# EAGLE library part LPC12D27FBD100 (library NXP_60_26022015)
LPC12D27 32-bit ARM Cortex-M0 microcontroller; 128 kB flash and 8 kB SRAM; 40 segment x 4 LCD driver AAL Eindhoven MK
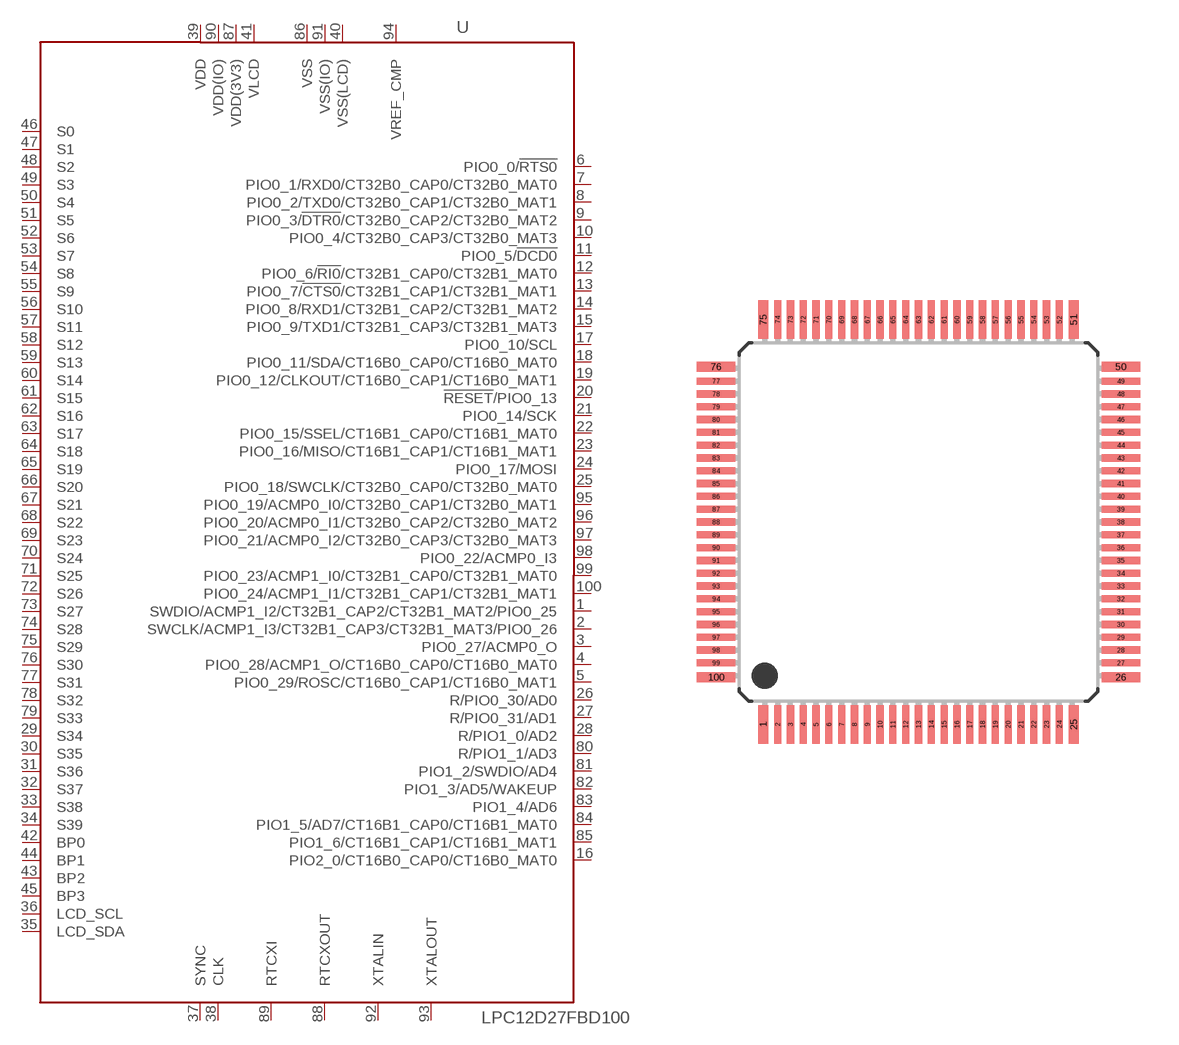
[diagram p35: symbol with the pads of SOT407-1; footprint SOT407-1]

Designator prefix U

## LPC12D27FBD100  [SOT407-1]
1  SWDIO/ACMP1_I2/CT32B1_CAP2/CT32B1_MAT2/PIO0_25
2  SWCLK/ACMP1_I3/CT32B1_CAP3/CT32B1_MAT3/PIO0_26
3  PIO0_27/ACMP0_O
4  PIO0_28/ACMP1_O/CT16B0_CAP0/CT16B0_MAT0
5  PIO0_29/ROSC/CT16B0_CAP1/CT16B0_MAT1
6  PIO0_0/!RTS0!
7  PIO0_1/RXD0/CT32B0_CAP0/CT32B0_MAT0
8  PIO0_2/TXD0/CT32B0_CAP1/CT32B0_MAT1
9  PIO0_3/!DTR0!/CT32B0_CAP2/CT32B0_MAT2
10  PIO0_4/CT32B0_CAP3/CT32B0_MAT3
11  PIO0_5/!DCD0!
12  PIO0_6/!RI0!/CT32B1_CAP0/CT32B1_MAT0
13  PIO0_7/!CTS0!/CT32B1_CAP1/CT32B1_MAT1
14  PIO0_8/RXD1/CT32B1_CAP2/CT32B1_MAT2
15  PIO0_9/TXD1/CT32B1_CAP3/CT32B1_MAT3
16  PIO2_0/CT16B0_CAP0/CT16B0_MAT0
17  PIO0_10/SCL
18  PIO0_11/SDA/CT16B0_CAP0/CT16B0_MAT0
19  PIO0_12/CLKOUT/CT16B0_CAP1/CT16B0_MAT1
20  !RESET!/PIO0_13
21  PIO0_14/SCK
22  PIO0_15/SSEL/CT16B1_CAP0/CT16B1_MAT0
23  PIO0_16/MISO/CT16B1_CAP1/CT16B1_MAT1
24  PIO0_17/MOSI
25  PIO0_18/SWCLK/CT32B0_CAP0/CT32B0_MAT0
26  R/PIO0_30/AD0
27  R/PIO0_31/AD1
28  R/PIO1_0/AD2
29  S34  out
30  S35  out
31  S36  out
32  S37  out
33  S38  out
34  S39  out
35  LCD_SDA
36  LCD_SCL
37  SYNC
38  CLK
39  VDD  pwr
40  VSS(LCD)  pwr
41  VLCD  pwr
42  BP0  out
43  BP2  out
44  BP1  out
45  BP3  out
46  S0  out
47  S1  out
48  S2  out
49  S3  out
50  S4  out
51  S5  out
52  S6  out
53  S7  out
54  S8  out
55  S9  out
56  S10  out
57  S11  out
58  S12  out
59  S13  out
60  S14  out
61  S15  out
62  S16  out
63  S17  out
64  S18  out
65  S19  out
66  S20  out
67  S21  out
68  S22  out
69  S23  out
70  S24  out
71  S25  out
72  S26  out
73  S27  out
74  S28  out
75  S29  out
76  S30  out
77  S31  out
78  S32  out
79  S33  out
80  R/PIO1_1/AD3
81  PIO1_2/SWDIO/AD4
82  PIO1_3/AD5/WAKEUP
83  PIO1_4/AD6
84  PIO1_5/AD7/CT16B1_CAP0/CT16B1_MAT0
85  PIO1_6/CT16B1_CAP1/CT16B1_MAT1
86  VSS  pwr
87  VDD(3V3)  pwr
88  RTCXOUT  pas
89  RTCXI  pas
90  VDD(IO)  pwr
91  VSS(IO)  pwr
92  XTALIN  pas
93  XTALOUT  pas
94  VREF_CMP  pwr
95  PIO0_19/ACMP0_I0/CT32B0_CAP1/CT32B0_MAT1
96  PIO0_20/ACMP0_I1/CT32B0_CAP2/CT32B0_MAT2
97  PIO0_21/ACMP0_I2/CT32B0_CAP3/CT32B0_MAT3
98  PIO0_22/ACMP0_I3
99  PIO0_23/ACMP1_I0/CT32B1_CAP0/CT32B1_MAT0
100  PIO0_24/ACMP1_I1/CT32B1_CAP1/CT32B1_MAT1

## Footprint SOT407-1 (pad centres in mm)
SOT407-1 LQFP100: plastic low profile quad flat package; 100 leads; body 14 x 14 x 1.4 mm JEDEC: MS-026 IEC: 136E20
smd 0.4 x 1.5: 1 -6.06,-7.9; 25 6.06,-7.9; 51 6.06,7.9; 75 -6.06,7.9
smd 0.28 x 1.5: 2 -5.5,-7.9; 3 -5,-7.9; 4 -4.5,-7.9; 5 -4,-7.9; 6 -3.5,-7.9; 7 -3,-7.9; 8 -2.5,-7.9; 9 -2,-7.9; 10 -1.5,-7.9; 11 -1,-7.9; 12 -0.5,-7.9; 13 0,-7.9; 14 0.5,-7.9; 15 1,-7.9; 16 1.5,-7.9; 17 2,-7.9; 18 2.5,-7.9; 19 3,-7.9; 20 3.5,-7.9; 21 4,-7.9; 22 4.5,-7.9; 23 5,-7.9; 24 5.5,-7.9; 52 5.5,7.9; 53 5,7.9; 54 4.5,7.9; 55 4,7.9; 56 3.5,7.9; 57 3,7.9; 58 2.5,7.9; 59 2,7.9; 60 1.5,7.9; 61 1,7.9; 62 0.5,7.9; 63 0,7.9; 64 -0.5,7.9; 65 -1,7.9; 66 -1.5,7.9; 67 -2,7.9; 68 -2.5,7.9; 69 -3,7.9; 70 -3.5,7.9; 71 -4,7.9; 72 -4.5,7.9; 73 -5,7.9; 74 -5.5,7.9
smd 1.5 x 0.4: 26 7.9,-6.06; 50 7.9,6.06; 76 -7.9,6.06; 100 -7.9,-6.06
smd 1.5 x 0.28: 27 7.9,-5.5; 28 7.9,-5; 29 7.9,-4.5; 30 7.9,-4; 31 7.9,-3.5; 32 7.9,-3; 33 7.9,-2.5; 34 7.9,-2; 35 7.9,-1.5; 36 7.9,-1; 37 7.9,-0.5; 38 7.9,0; 39 7.9,0.5; 40 7.9,1; 41 7.9,1.5; 42 7.9,2; 43 7.9,2.5; 44 7.9,3; 45 7.9,3.5; 46 7.9,4; 47 7.9,4.5; 48 7.9,5; 49 7.9,5.5; 77 -7.9,5.5; 78 -7.9,5; 79 -7.9,4.5; 80 -7.9,4; 81 -7.9,3.5; 82 -7.9,3; 83 -7.9,2.5; 84 -7.9,2; 85 -7.9,1.5; 86 -7.9,1; 87 -7.9,0.5; 88 -7.9,0; 89 -7.9,-0.5; 90 -7.9,-1; 91 -7.9,-1.5; 92 -7.9,-2; 93 -7.9,-2.5; 94 -7.9,-3; 95 -7.9,-3.5; 96 -7.9,-4; 97 -7.9,-4.5; 98 -7.9,-5; 99 -7.9,-5.5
